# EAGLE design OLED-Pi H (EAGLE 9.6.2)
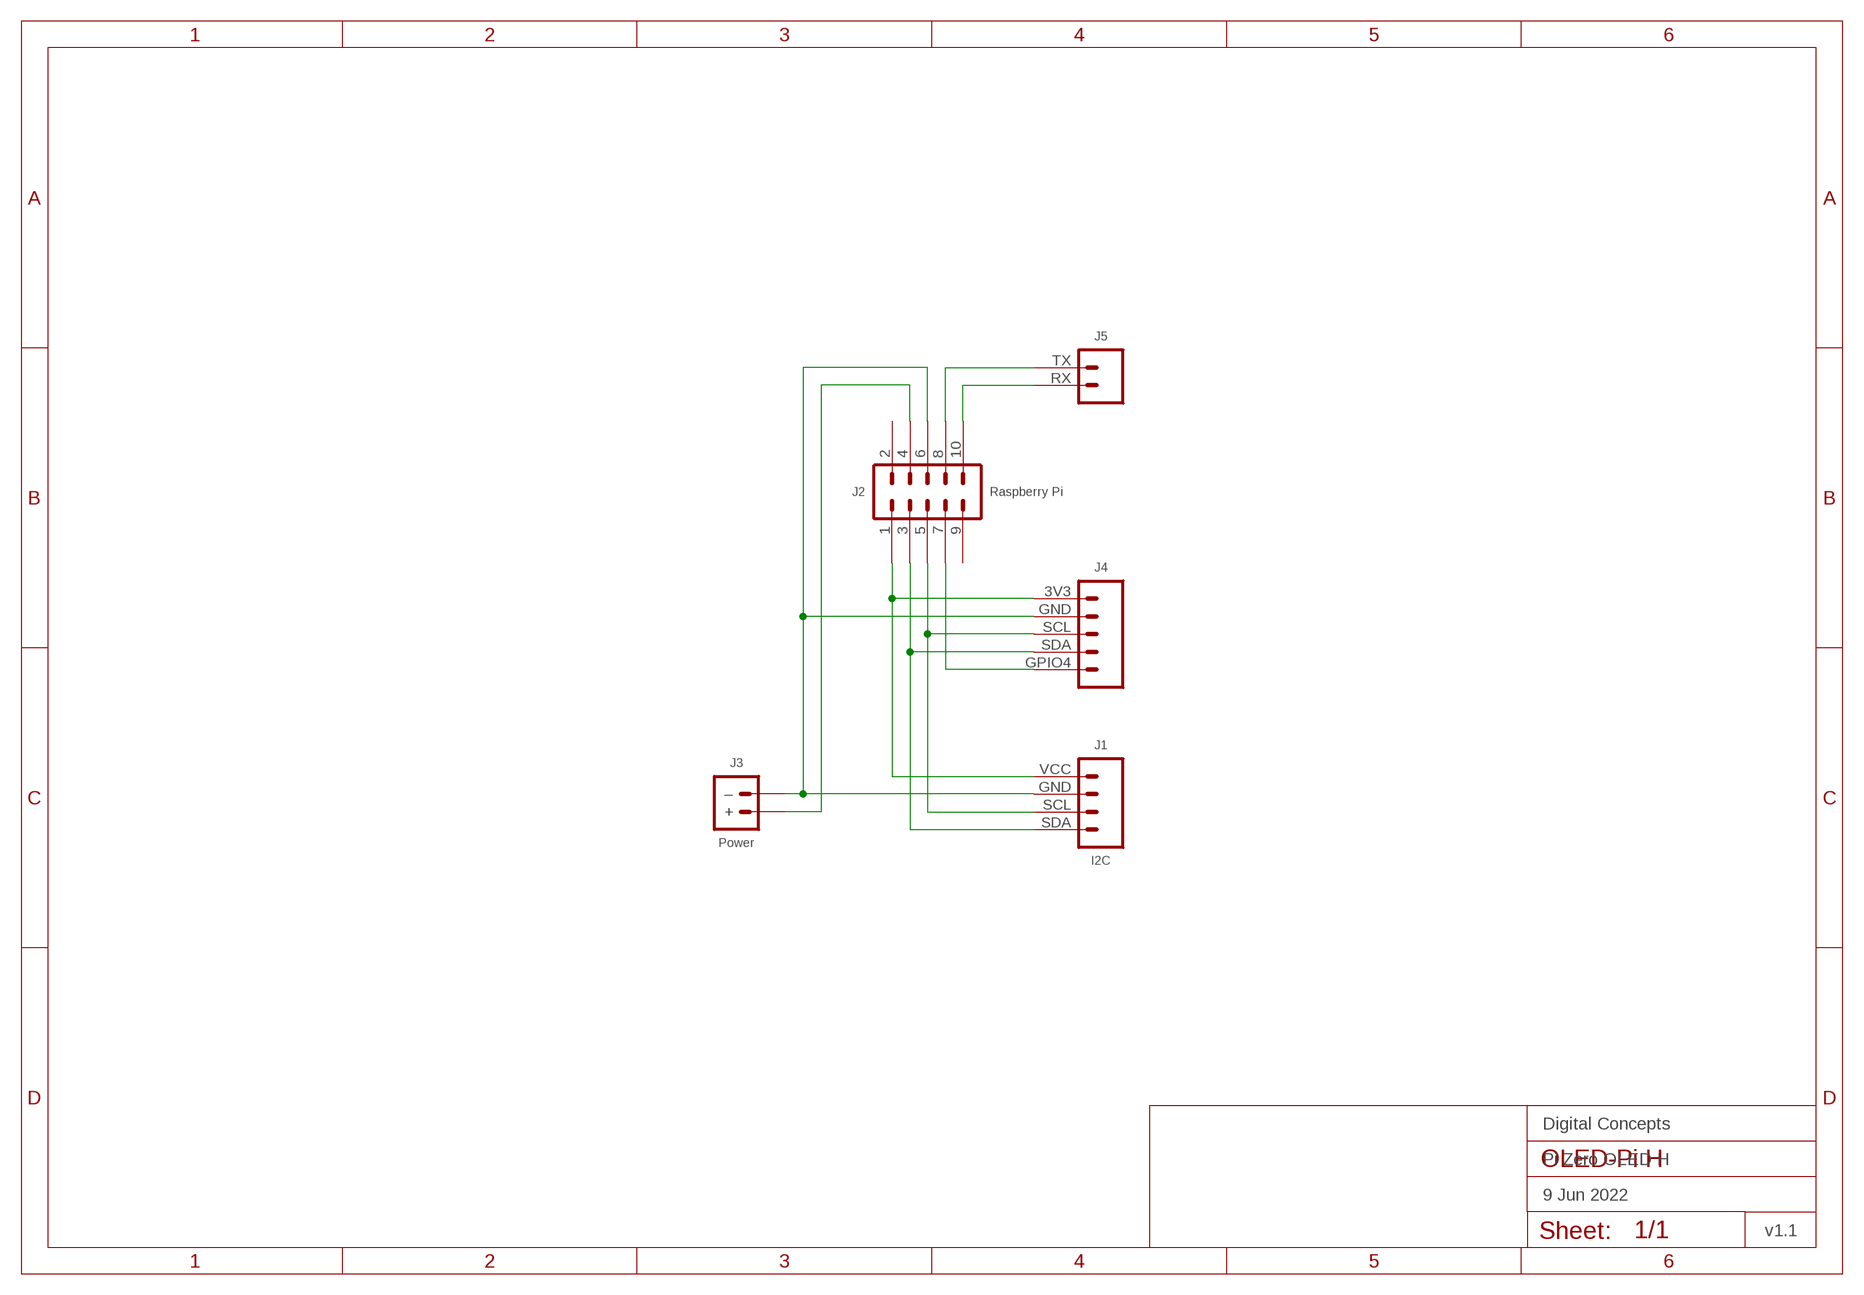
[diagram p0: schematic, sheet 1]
FRAME1 (FRAME-A4L-LOC): DATE: 9 Jun 2022; OWNER: Digital Concepts; TITLE: Pi Zero OLED H; VERSION: v1.1

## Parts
J1  I2C  HEADER-1X4-I2C  [CONN_04-I2C]
J2  Raspberry Pi  HEADER-2X5-PI-1  [CONN_2X5-PI-1]
J3  Power  JST-PH2.0-2-HORIZONTAL-POWERJST-PTH-2  [JST-PH2.0-2-HORIZONTAL-POWER]
J4  JST-PH2.0-5-HORIZONTAL-OLED-PI  [JST-PH2.0-5-HORIZONTAL-OLED-PI]
J5  JST-PH2.0-2-HORIZONTAL-TX-RXJST-PTH-2  [JST-PH2.0-2-HORIZONTAL=TX-RX]

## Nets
N$1: J1.GND J2.6 J3.-(–) J4.GND
N$2: J2.4 J3.+
N$3: J1.VCC J2.1 J4.3V3
N$4: J1.SDA J2.3 J4.SDA
N$5: J1.SCL J2.5 J4.SCL
N$6: J2.7 J4.GPIO4
N$7: J2.10 J5.RX
N$8: J2.8 J5.TX
Unconnected: J2.2 J2.9

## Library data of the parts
J1 = digitalconcepts:HEADER-1X4-I2C: I2C Interface [Pin 1 Vcc] 4-Pin Header
J2 = digitalconcepts:HEADER-2X5-PI-1: Ras-Pi 2x5 PTH Header Rapsberry Pi, starting at Pin 1
J3 = digitalconcepts:JST-PH2.0-2-HORIZONTAL-POWER: PH2.0 2P Right Angle PCB Connector; PROD_ID: CONN-09863; SKU: PRT-09914
J4 = digitalconcepts:JST-PH2.0-5-HORIZONTAL-OLED-PI: PH2.0 5P OLED-Pi Horizontal Connector
J5 = digitalconcepts:JST-PH2.0-2-HORIZONTAL-TX-RX: PH2.0 2P Right Angle PCB Connector with Tx/Rx Pin Labels; PROD_ID: CONN-09863; SKU: PRT-09914

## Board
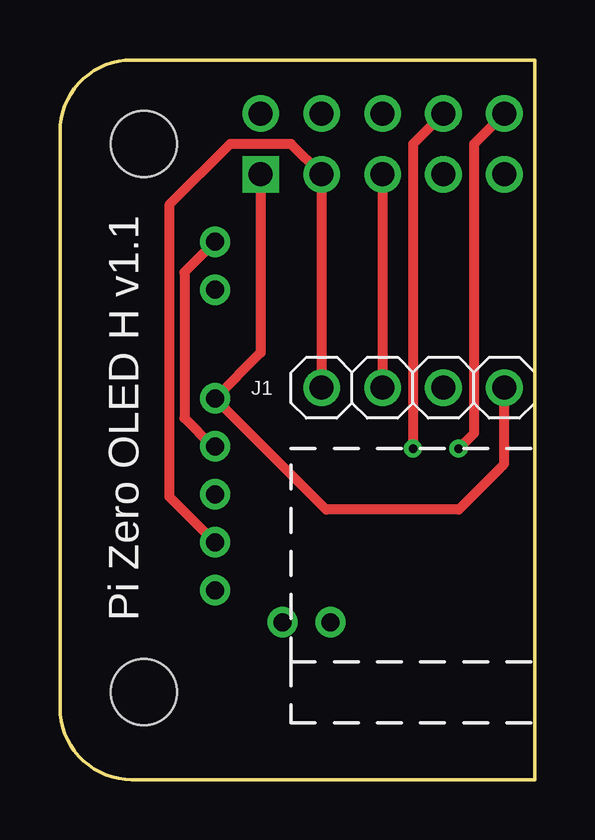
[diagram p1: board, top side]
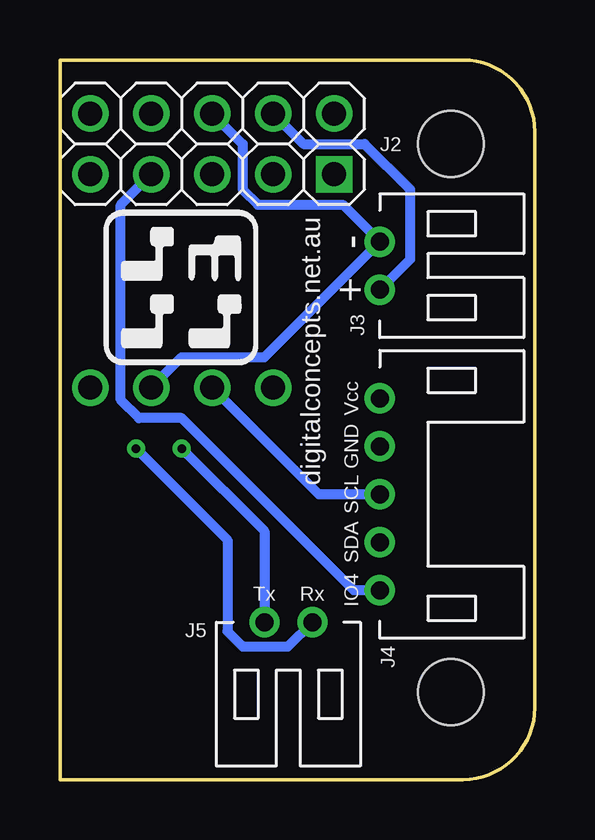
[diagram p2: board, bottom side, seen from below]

Size 19.8 x 30 mm. Coordinates in mm from the lower left corner, seen from the top.
Outline: 19.8,30 19.8,0 2.99,0 arc-90 0,2.99 0,27.01 arc-90 2.99,30 19.8,30
Copper layers (1*16): Top 0.035mm / dielectric 1.5mm / Bottom 0.035mm
Design rules "default *": minimum track width 6mil, minimum drill 0.35mm, track to track 6mil, track to pad 6mil, pad to pad 6mil, via to via 6mil, smd to smd 6mil, copper to edge 6mil, drill to drill 6mil, minimum pad ring 10mil, minimum via ring 8mil, stop-mask expansion 4mil, vias tented up to drill 0mil, thermal gap 10mil
Holes 2.75 mm at 3.5,26.5 3.5,3.64

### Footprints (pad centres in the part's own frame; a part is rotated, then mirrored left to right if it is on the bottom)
CONN_04-I2C = drill 1 pad 1.524: GND 2.54,0; SCL 5.08,0; SDA 7.62,0; VCC 0,0
CONN_2X5-PI-1 = drill 1 pad 1.524 square: 1 0,0 | drill 1 pad 1.524: 2 0,2.54; 3 2.54,0; 4 2.54,2.54; 5 5.08,0; 6 5.08,2.54; 7 7.62,0; 8 7.62,2.54; 9 10.16,0; 10 10.16,2.54
JST-PH2.0-2-HORIZONTAL-POWER = drill 0.75: + 1,0; - -1,0
JST-PH2.0-5-HORIZONTAL-OLED-PI = drill 0.75: 3V3 4,0; GND 2,0; GPIO4 -4,0; SCL 0,0; SDA -2,0
JST-PH2.0-2-HORIZONTAL=TX-RX = drill 0.75: RX -1,0; TX 1,0

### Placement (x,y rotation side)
J1  18.53,16.34 180 top
J2  8.37,25.23 0 top
J3  6.47,21.42 270 bottom
J4  6.47,11.89 90 bottom
J5  10.28,6.56 180 bottom

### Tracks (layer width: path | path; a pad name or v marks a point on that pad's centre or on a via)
N$1
  Top 0.406: J3.- 5.2,21.15 5.2,15.07 6.37,13.89 J4.GND
  Bottom 0.406: J2.6 12.18,26.5 12.18,24.59 11.55,23.96 8.01,23.96 J3.- 11.28,17.61 14.72,17.61 J1.GND
N$2
  Bottom 0.406: J3.+ 5.2,21.69 5.2,24.59 7.1,26.5 9.64,26.5 J2.4
N$3
  Top 0.406: J1.VCC 18.53,13.16 16.63,11.26 11.1,11.26 J4.3V3 8.37,17.8 J2.1
N$4
  Top 0.406: J1.SDA J2.3 9.64,26.5 7.1,26.5 4.56,23.96 4.56,11.8 J4.SDA
N$5
  Top 0.406: J2.5 J1.SCL
  Bottom 0.406: J1.SCL 9.01,11.89 J4.SCL
N$6
  Bottom 0.406: J4.GPIO4 7.55,7.89 14.72,15.07 16.5,15.07 17.26,15.83 17.26,23.96 J2.7
N$7  (via drill 0.35)
  Top 0.406: J2.10 17.26,26.5 17.26,14.43 v16.63,13.8
  Bottom 0.406: v16.63,13.8 12.82,9.99 12.82,6.18 12.18,5.54 10.29,5.54 J5.RX
N$8  (via drill 0.35)
  Top 0.406: J2.8 14.72,26.5 v14.72,13.8
  Bottom 0.406: v14.72,13.8 11.28,10.35 J5.TX

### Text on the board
tPlace: Pi Zero OLED H v1.1
bPlace: digitalconcepts.net.au
bNames: Vcc | GND | SCL | SDA | IO4 | Rx | Tx
tValues: SDA | SCL | GND | VCC
bValues: 5V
